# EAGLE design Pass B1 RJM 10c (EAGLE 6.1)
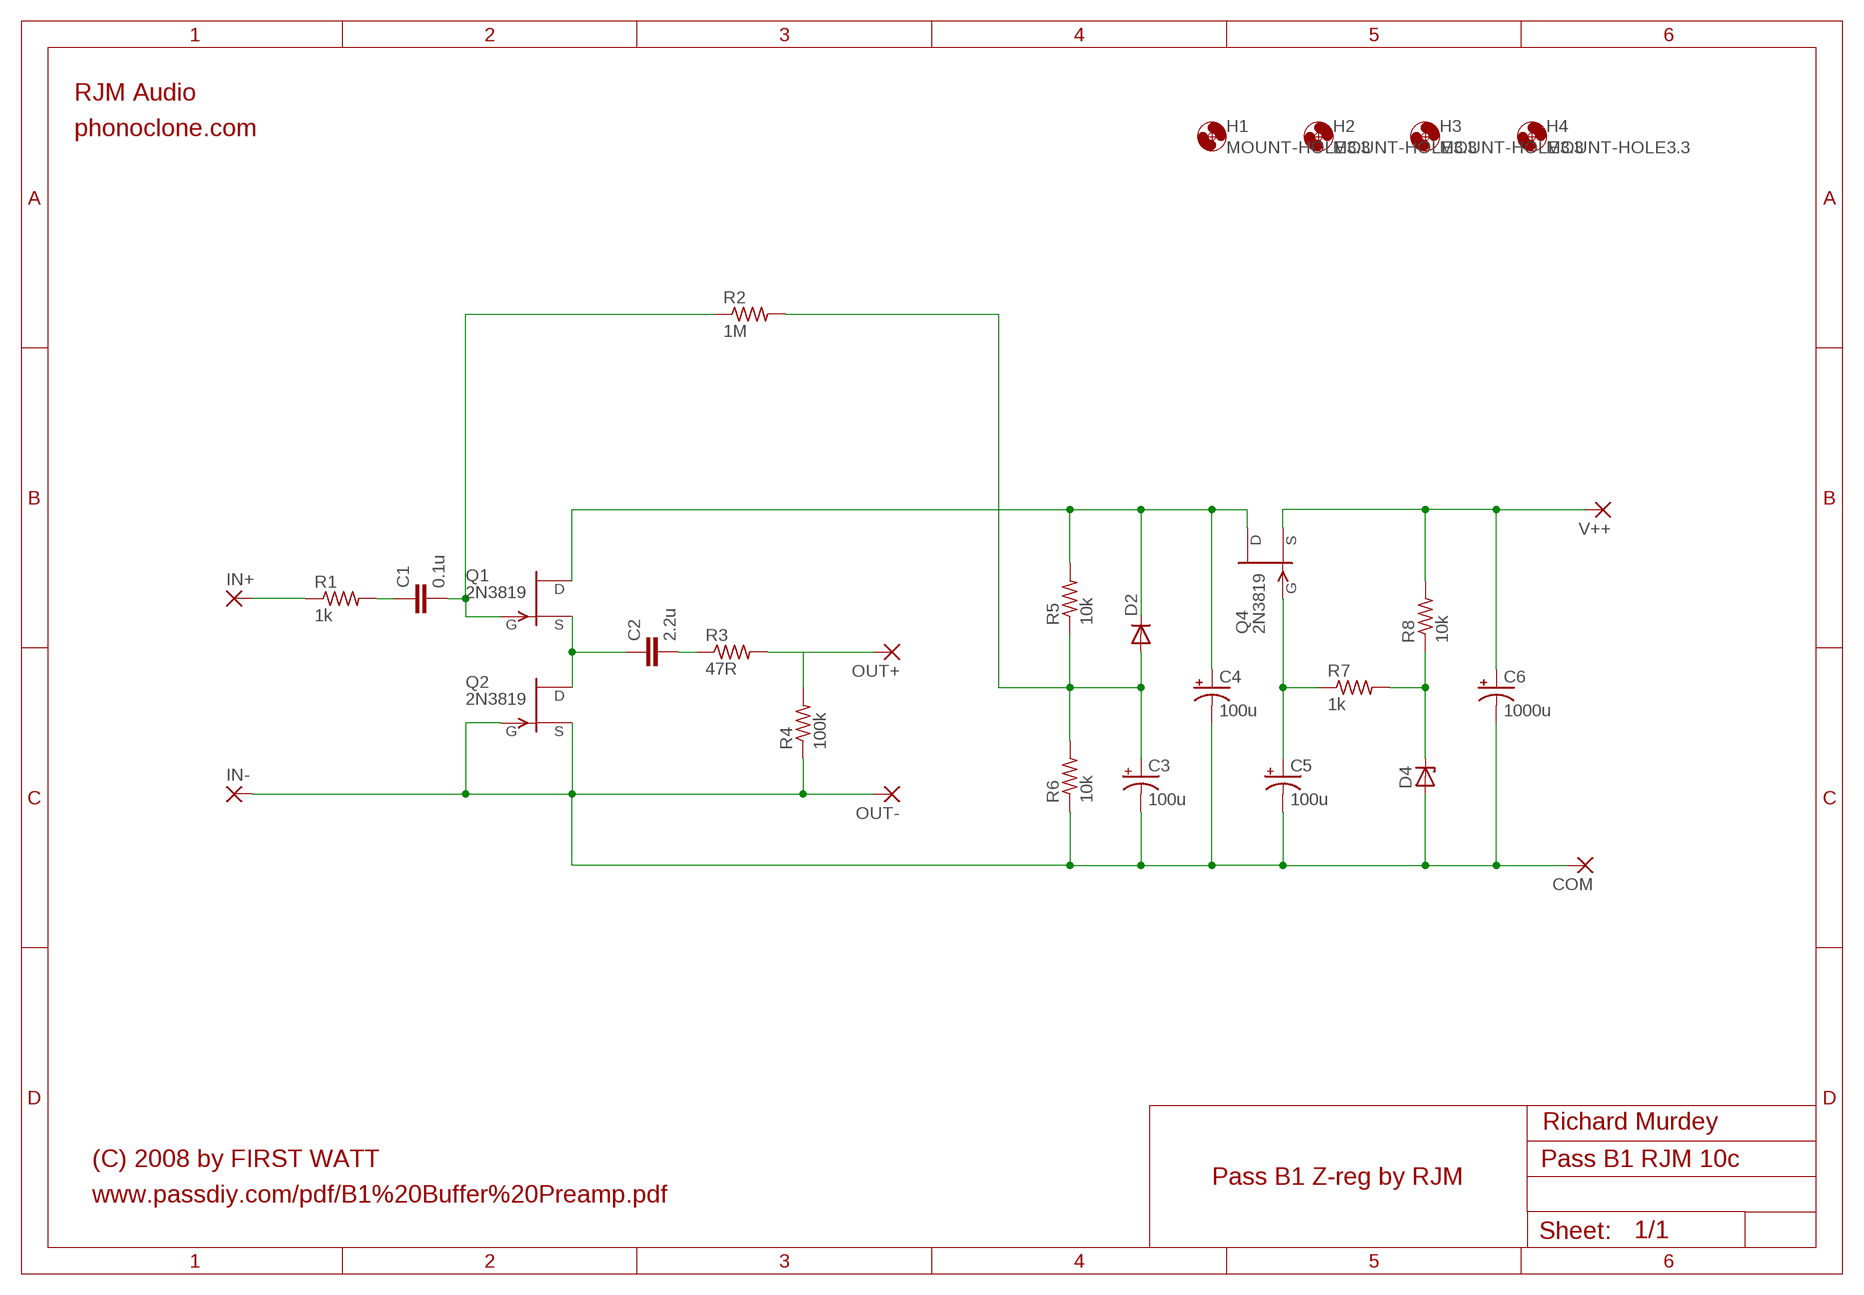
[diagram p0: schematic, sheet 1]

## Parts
C1  0.1u  C-EU050-050X075  [C050-050X075]
C2  2.2u  C-EU225-108X268  [C225-108X268]
C3  100u  CPOL-USE5-6  [E5-6]
C4  100u  CPOL-USE5-6  [E5-6]
C5  100u  CPOL-USE5-6  [E5-6]
C6  1000u  CPOL-USE5-10.5  [E5-10,5]
COM  2,54/1,1  [2,54/1,1]
D2  1N4004  [DO41-10]
D4  BZX85  [DO41Z10]
H1  MOUNT-HOLE3.3  [3,3]
H2  MOUNT-HOLE3.3  [3,3]
H3  MOUNT-HOLE3.3  [3,3]
H4  MOUNT-HOLE3.3  [3,3]
IN+  2,54/1,1  [2,54/1,1]
IN-  2,54/1,1  [2,54/1,1]
OUT+  2,54/1,1  [2,54/1,1]
OUT-  2,54/1,1  [2,54/1,1]
Q1  2N3819  [TO92]
Q2  2N3819  [TO92]
Q4  2N3819  [TO92]
R1  1k  R-US_0309/12  [0309/12]
R2  1M  R-US_0309/12  [0309/12]
R3  47R  R-US_0309/12  [0309/12]
R4  100k  R-US_0309/12  [0309/12]
R5  10k  R-US_0309/12  [0309/12]
R6  10k  R-US_0309/12  [0309/12]
R7  1k  R-US_0309/12  [0309/12]
R8  10k  R-US_0309/12  [0309/12]
V++  2,54/1,1  [2,54/1,1]

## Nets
BIASA: C3.+ D2.A R2.2 R5.1 R6.2
BIASB: C1.2 Q1.2(G) R2.1
COM: C3.- C4.- C5.- C6.- COM.1(P) D4.A IN-.1(P) OUT-.1(P) Q2.2(G) Q2.3(S) R4.1 R6.1
INPUT: IN+.1(P) R1.1
N$2: C1.1 R1.2
N$6: C2.1 Q1.3(S) Q2.1(D)
N$9: C2.2 R3.1
N$10: OUT+.1(P) R3.2 R4.2
N$37: D4.C R7.2 R8.1
N$39: C5.+ Q4.2(G) R7.1
V+: C4.+ D2.C Q1.1(D) Q4.1(D) R5.2
V++: C6.+ Q4.3(S) R8.2 V++.1(P)

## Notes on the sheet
- RJM Audio
- phonoclone.com
- Richard Murdey
- (C) 2008 by FIRST WATT
- Pass B1 Z-reg by RJM
- www.passdiy.com/pdf/B1%20Buffer%20Preamp.pdf

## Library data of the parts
C1 C2 = resistor:C-EU: CAPACITOR, European symbol
C3-C6 = resistor:CPOL-US: POLARIZED CAPACITOR, American symbol
COM IN+ IN- OUT+ OUT- V++ = wirepad:2,54/1,1: THROUGH-HOLE PAD
D2 = diode:1N4004: DIODE
D4 = diode:BZX85: Z DIODE
H1-H4 = holes:MOUNT-HOLE: MOUNTING HOLE with drill center marker
Q1 Q2 Q4 = transistor-fet:2N3819: N-Channel Junction FET
R1-R8 = resistor:R-US_: RESISTOR, American symbol

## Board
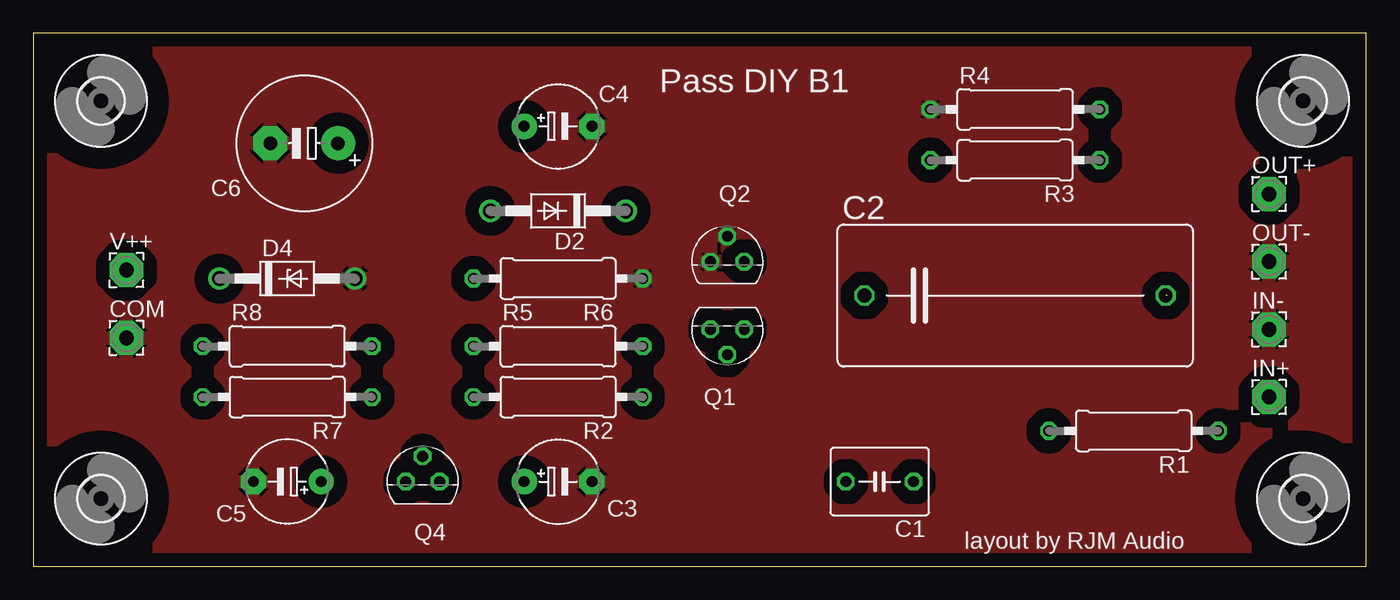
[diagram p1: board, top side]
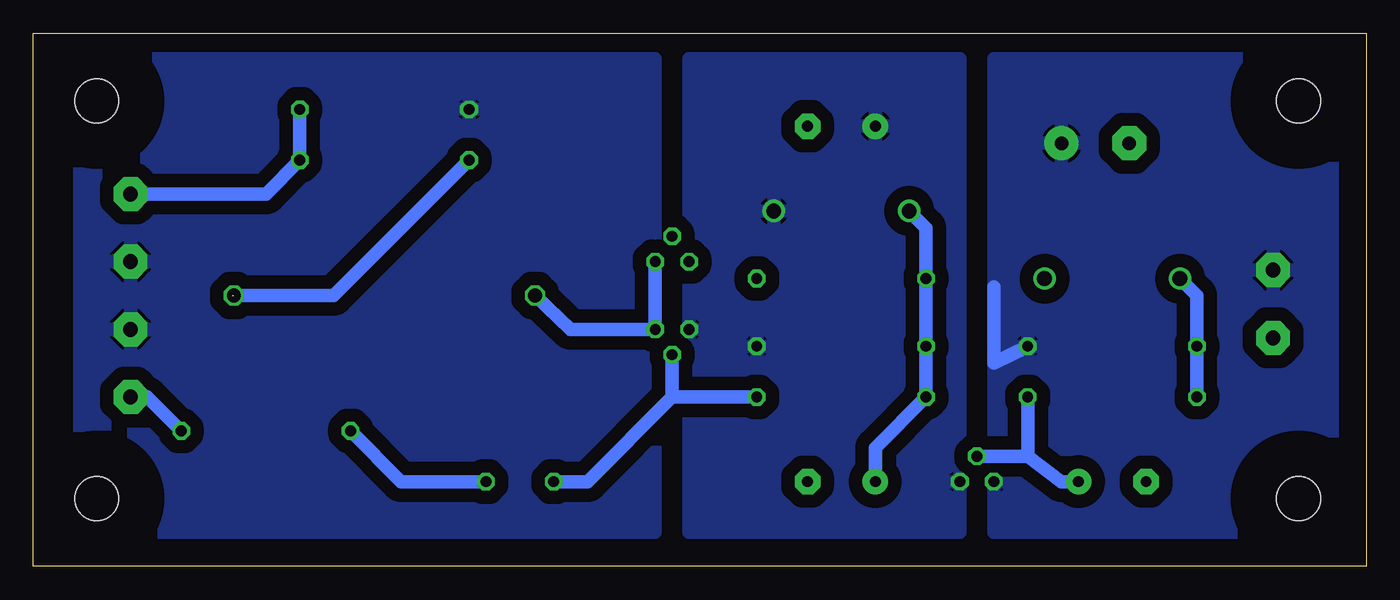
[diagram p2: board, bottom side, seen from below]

Size 100 x 40 mm. Coordinates in mm from the lower left corner, seen from the top.
Outline: 0,0 100,0 100,40 0,40 0,0
Copper layers (1*16): Top 0.035mm / dielectric 1.5mm / Bottom 0.035mm
Design rules: minimum track width 10mil, minimum drill 24mil, track to track 8mil, track to pad 8mil, pad to pad 8mil, via to via 8mil, smd to smd 8mil, copper to edge 40mil, drill to drill 8mil, minimum pad ring 10mil, minimum via ring 8mil, stop-mask expansion 4mil, vias tented up to drill 0mil, thermal gap 10mil

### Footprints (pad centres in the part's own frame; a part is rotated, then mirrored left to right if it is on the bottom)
C050-050X075 = drill 0.813 octagon: 1 -2.54,0; 2 2.54,0
C225-108X268 = drill 1.016 octagon: 1 -11.303,0; 2 11.303,0
E5-6 = drill 0.813 pad 1.905: + -2.54,0 | drill 0.813 pad 1.905 octagon: - 2.54,0
E5-10,5 = drill 1.016 pad 2.54: + -2.54,0 | drill 1.016 pad 2.54 octagon: - 2.54,0
2,54/1,1 = drill 1.118 pad 2.54 octagon: 1 0,0
DO41-10 = drill 1.118: A 5.08,0; C -5.08,0
DO41Z10 = drill 1.118: A 5.08,0; C -5.08,0
3,3 = hole 3.3: 0,0
TO92 = drill 0.813 octagon: 1 1.27,0; 2 0,1.905; 3 -1.27,0
0309/12 = drill 0.813 octagon: 1 -6.35,0; 2 6.35,0

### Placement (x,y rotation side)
C1  63.5,6.35 180 top
C2  73.66,20.32 0 top
C3  39.37,6.35 0 top
C4  39.37,33.02 0 top
C5  19.05,6.35 180 top
C6  20.32,31.75 180 top
COM  6.99,17.14 0 top
D2  39.37,26.67 180 top
D4  19.05,21.59 0 top
H1  5.08,5.08 0 top
H2  5.08,34.92 0 top
H3  95.25,34.92 0 top
H4  95.25,5.08 0 top
IN+  92.71,12.7 0 top
IN-  92.71,17.78 0 top
OUT+  92.71,27.94 0 top
OUT-  92.71,22.86 0 top
Q1  52.07,17.78 180 top
Q2  52.07,22.86 0 top
Q4  29.21,6.35 0 top
R1  82.55,10.16 180 top
R2  39.37,12.7 180 top
R3  73.66,30.48 0 top
R4  73.66,34.29 0 top
R5  39.37,16.51 0 top
R6  39.37,21.59 180 top
R7  19.05,12.7 180 top
R8  19.05,16.51 0 top
V++  6.99,22.23 0 top

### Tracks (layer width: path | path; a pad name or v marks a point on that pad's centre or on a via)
BIASA
  Bottom 1.016: D2.A 33.02,25.4 R6.2 R5.1 R2.2 36.83,8.89 C3.+
BIASB
  Bottom 1.016: Q1.2 52.07,12.7 | 52.07,12.7 R2.1 | 52.07,12.7 58.42,6.35 C1.2
COM
  pour Top (isolate 1.016): 2.54,2.54 2.54,36.83 99.06,36.83 99.06,2.54
  pour Bottom (isolate 1.016, rank 3): 53.34,2.54 53.34,38.1 96.52,38.1 96.52,2.54
COM2
  pour Top (isolate 1.016): 0,40.64 0,0 100.33,0 100.33,40.64
INPUT
  Bottom 1.016: R1.1 91.44,12.7 IN+.1
N$2
  Bottom 1.016: C1.1 72.39,6.35 R1.2
N$6
  Bottom 1.016: Q2.1 Q1.3 59.69,17.78 C2.1
N$9  (1 unrouted)
  Bottom 1.016: R3.1 77.47,20.32 85.09,20.32
N$10
  Bottom 1.016: R4.2 R3.2 82.55,27.94 OUT+.1
N$37
  Bottom 1.016: R7.2 R8.1 12.7,20.32 D4.C
N$39
  Bottom 1.016: C5.+ 22.86,6.35 25.4,8.26 | 25.4,8.26 R7.1 | Q4.2 25.4,8.26
V+
  pour Bottom (isolate 1.016, rank 2): 30.48,2.54 30.48,38.1 50.8,38.1 50.8,2.54
V++
  Bottom 1.016: 27.94,20.95 27.94,15.24 R8.2
  pour Bottom (isolate 1.016): 2.54,38.1 27.94,38.1 27.94,2.54 2.54,2.54

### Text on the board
tPlace: Pass DIY B1 | layout by RJM Audio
